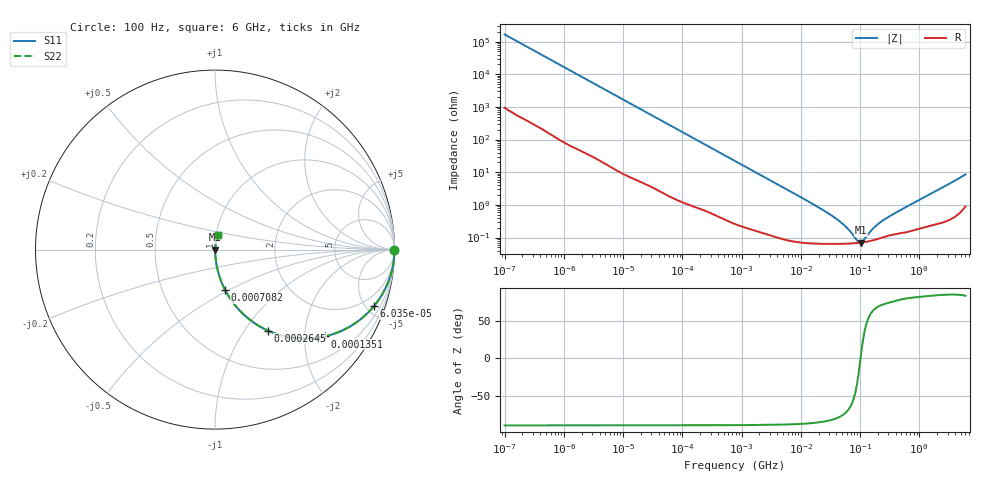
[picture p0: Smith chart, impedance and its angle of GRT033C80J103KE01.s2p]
!Murata Part Number: GRT033C80J103KE01
!These Parameters are Measured in Series Mode Connection
!Data Generated on Jun 19, 2026
!  o--ll--o
!Port1  Port2
!  o------o
!Operation Temp=25[degC], DC Bias Voltage=0[V]
!Freq. Start=100[Hz] Stop=6[GHz] 401[Steps]
# Hz S RI R 50
!Freq.(Hz) S11(Real) S11(Imag) S21(Real) S21(Imag) S12(Real) S12(Imag) S22(Real) S22(Imag)
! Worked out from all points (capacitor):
!   401 points, 100 Hz to 6 GHz, reference 50 ohm
!   read as one part in series: C = 9.61 nF near 109 Hz
!   lowest |Z| = 70 mohm at 102 MHz (marker M1)
!   series resonance near 101.8 MHz, so ESL is about 250 pH
!   S11 on the Smith chart (normalised r, x): 100 Hz: open; 60.35 kHz: 1.04, -5.60; 135.1 kHz: 1.02, -2.51; 264.5 kHz: 1.01, -1.29; 708.2 kHz: 1.01, -0.48; 6 GHz: 1.02, +0.17
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100  1 -0.000605  3.8e-06 0.000605  3.8e-06 0.000605  1 -0.000605
2008  0.9998 -0.012  0.000208 0.012  0.000208 0.012  0.9998 -0.012
12041  0.9945 -0.0713  0.0055 0.0713  0.0055 0.0713  0.9945 -0.0713
40335  0.9446 -0.2255  0.0554 0.2255  0.0554 0.2255  0.9446 -0.2255
60352  0.8853 -0.3155  0.1147 0.3155  0.1147 0.3155  0.8853 -0.3155
90302  0.7767 -0.413  0.2233 0.413  0.2233 0.413  0.7767 -0.413
135116  0.6105 -0.4838  0.3895 0.4838  0.3895 0.4838  0.6105 -0.4838
184852  0.4577 -0.4939  0.5423 0.4939  0.5423 0.4939  0.4577 -0.4939
264476  0.2943 -0.451  0.7057 0.451  0.7057 0.451  0.2943 -0.451
413847  0.1478 -0.3497  0.8522 0.3497  0.8522 0.3497  0.1478 -0.3497
708247  0.0574 -0.227  0.9426 0.227  0.9426 0.227  0.0574 -0.227
774597  0.0488 -0.2096  0.9512 0.2096  0.9512 0.2096  0.0488 -0.2096
2594782  0.00566 -0.066  0.9943 0.066  0.9943 0.066  0.00566 -0.066
1.555665e7  0.000778 -0.0109  0.9992 0.0109  0.9992 0.0109  0.000778 -0.0109
4.556224e7  0.000652 -0.00305  0.9993 0.00305  0.9993 0.00305  0.000652 -0.00305
6.233367e7  0.000657 -0.00174  0.9993 0.00174  0.9993 0.00174  0.000657 -0.00174
8.918374e7  0.000682 -0.000452  0.9993 0.000452  0.9993 0.000452  0.000682 -0.000452
1.020051e8  0.0007 5.4e-06  0.9993 -5.4e-06  0.9993 -5.4e-06  0.0007 5.4e-06
1.166697e8  0.000723 0.000461  0.9993 -0.000461  0.9993 -0.000461  0.000723 0.000461
1.825626e8  0.000868 0.00205  0.9991 -0.00205  0.9991 -0.00205  0.000868 0.00205
3.124326e8  0.00118 0.00429  0.9988 -0.00429  0.9988 -0.00429  0.00118 0.00429
6e9  0.016 0.083  0.984 -0.083  0.984 -0.083  0.016 0.083
